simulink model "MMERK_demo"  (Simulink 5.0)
settings: Solver=ode45  StartTime=0.0  StopTime=100.0  RelTol=1e-3

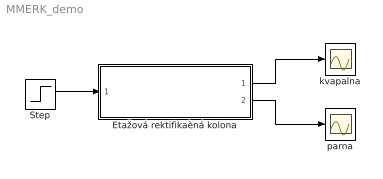
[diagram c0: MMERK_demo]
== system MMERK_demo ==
  Etažová rektifikaèná kolona : Subsystem  mask(ETAZOVA REKTIFIKACNA KOLONA){vst=[0 0 1 0 0 0], por=[0 0 0 0 0 0], N=6, F=4, axb=[-5.1346083  15.131084  46.224365e-6  -16.30502  25.2741], nii=[60 100], parF=[0.234 0.5], par1=[0.165 -1], par2=[0.16 -1], H=[0.2 1], vystup=[1 1 0 0 1 0 0 1]}
      mask prompts: vst "Riadiace - akèné velièiny    ano-1  nie-0    [nF xF nL nD nV nW]"; por "Poruchové velièiny   ano-1  nie-0    [nF xF nD nL nV nW]"; N "Poèet etáži"; F "Nástreková etáž"; axb "Konštanty rovnovážnej krivky   y=(ax^2+bx+c)/(dx^2+ex+1)"; nii "Uèinnosti     [jednotlivé etáže   varák]"; parF "Tok látkového množstva a molový zlomok nástreku    [nF  xF]"; par1 "Tok látkového množstva destilátu a destil. zvyšku  [nD nW]"; par2 "Tok látkového množstva spätného toku a odchádzajúcich pár   [nL  nV]"; H "Zádrže kvapaliny  [jednotlivé etáže   varák]"; vystup "Výstupné velièiny   xi-yi     1 - ano    0 - nie    [.. xi-yi ..]"
      mask help: Etážová rektifikaèná kolona - nelineárny model
      mask init:
      | nF=parF(1);
      | xF=parF(2);
      | nD=par1(1);
      | nW=par1(2);
      | nL=par2(1);
      | nV=par2(2);
      | C=kolona4(N,vystup);
  Step : Step  Time=0  Before=0.16  After=0.16  SampleTime=0
  kvapalna : Scope
  parna : Scope
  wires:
  Step/1 -> Etažová rektifikaèná kolona/1(In1)
  Etažová rektifikaèná kolona/1(Out1) -> kvapalna/1
  Etažová rektifikaèná kolona/2(Out2) -> parna/1

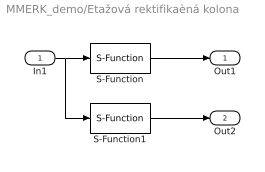
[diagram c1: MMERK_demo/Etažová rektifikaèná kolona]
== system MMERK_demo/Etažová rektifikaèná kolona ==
  In1 : Inport
  S-Function : S-Function  FunctionName=kolona_x  Parameters=N,F,axb,nii,nF,xF,nD,nL,nV,nW,H,C,vst,por
  S-Function1 : S-Function  FunctionName=kolona_y  Parameters=N,F,axb,nii,nF,xF,nD,nL,nV,nW,H,C,vst,por
  Out1 : Outport
  Out2 : Outport  Port=2
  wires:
  S-Function/1 -> Out1/1
  In1/1 -> S-Function/1, S-Function1/1
  S-Function1/1 -> Out2/1
